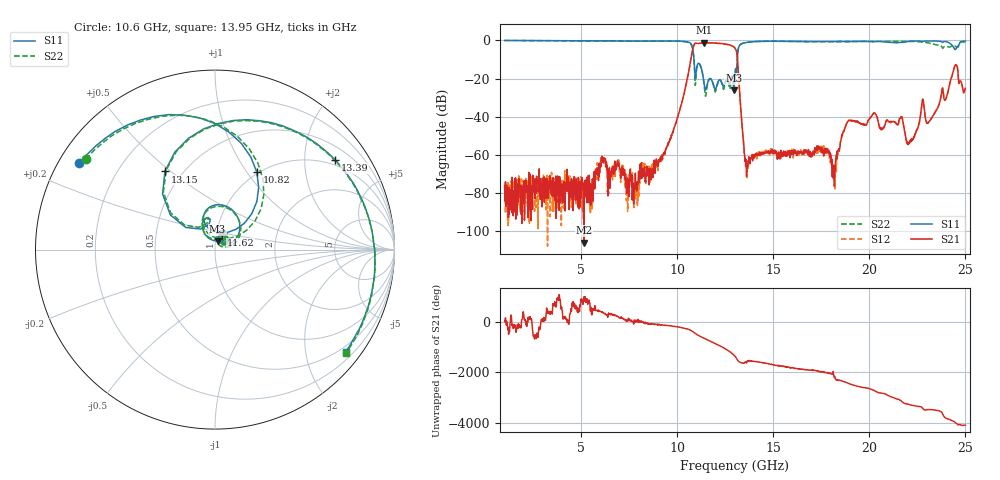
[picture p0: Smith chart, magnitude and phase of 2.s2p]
!The following data was pulled from an Agilent PNA
!This sNp file was generated from the data in the RF Test software
!NOTE:  Smoothing/Math/Corrections applied on any given trace ARE included in the data saved here
# MHz S dB R 50
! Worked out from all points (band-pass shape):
!   1601 points, 1 GHz to 25 GHz, reference 50 ohm
!   highest |S21| = -1.19 dB at 11.41 GHz (marker M1); lowest = -106.1 dB at 5.14 GHz (marker M2)
!   |S21| within 3 dB of the highest: 10.81 GHz to 13.01 GHz (2.2 GHz wide, 18.5 % of centre)
!   lowest |S11| = -26.2 dB at 12.94 GHz (marker M3), VSWR 1.10, Z = 51.2 + j4.84 ohm
!   |S11| at or under -10 dB: 10.86 GHz to 13.12 GHz (2.257 GHz wide, 18.8 % of centre)
!   |S22| runs from -29.3 to 0.0 dB; largest |S21 - S12| = 0.013
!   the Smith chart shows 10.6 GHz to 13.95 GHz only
!   S11 on the Smith chart (normalised r, x): 10.6 GHz: 0.06, +0.29; 10.82 GHz: 0.98, +1.11; 11.62 GHz: 1.06, +0.18; 13.15 GHz: 0.40, +0.48; 13.39 GHz: 0.84, +2.78; 13.95 GHz: 0.36, -2.86
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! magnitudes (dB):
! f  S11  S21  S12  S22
! 1 GHz  0.0  -76.2  -81.3  0.0
! 5.005 GHz  -0.2  -72.9  -79.2  -0.3
! 5.14 GHz  -0.2  -106.1  -79.2  -0.3
! 6.1 GHz  -0.3  -63.4  -63.9  -0.4
! 9.01 GHz  -0.3  -62.7  -64.8  -0.3
! 10.6 GHz  -1.0  -15.8  -15.8  -1.1
! 10.82 GHz  -6.2  -3.5  -3.5  -6.4
! 11.41 GHz  -23.8  -1.2  -1.1  -25.2
! 11.62 GHz  -20.8  -1.3  -1.3  -21.2
! 12.94 GHz  -26.2  -3.4  -3.4  -24.9
! 13 GHz  -17.3  -4.1  -4.1  -17.3
! 13.15 GHz  -5.7  -13.0  -13.1  -5.7
! 13.39 GHz  -1.6  -47.1  -47.1  -1.6
! 13.6 GHz  -1.1  -71.5  -64.2  -1.1
! 13.95 GHz  -0.7  -60.8  -60.6  -0.6
! 17 GHz  -0.6  -61.0  -59.2  -0.7
! 18.16 GHz  -0.6  -71.0  -73.3  -0.7
! 18.93 GHz  -0.6  -41.9  -42.1  -0.6
! 21.01 GHz  -0.9  -42.6  -43.1  -0.4
! 22.07 GHz  -0.5  -54.0  -53.4  -0.5
! 24.46 GHz  -4.8  -13.2  -13.1  -2.9
! 25 GHz  -0.4  -25.1  -25.2  -0.9
